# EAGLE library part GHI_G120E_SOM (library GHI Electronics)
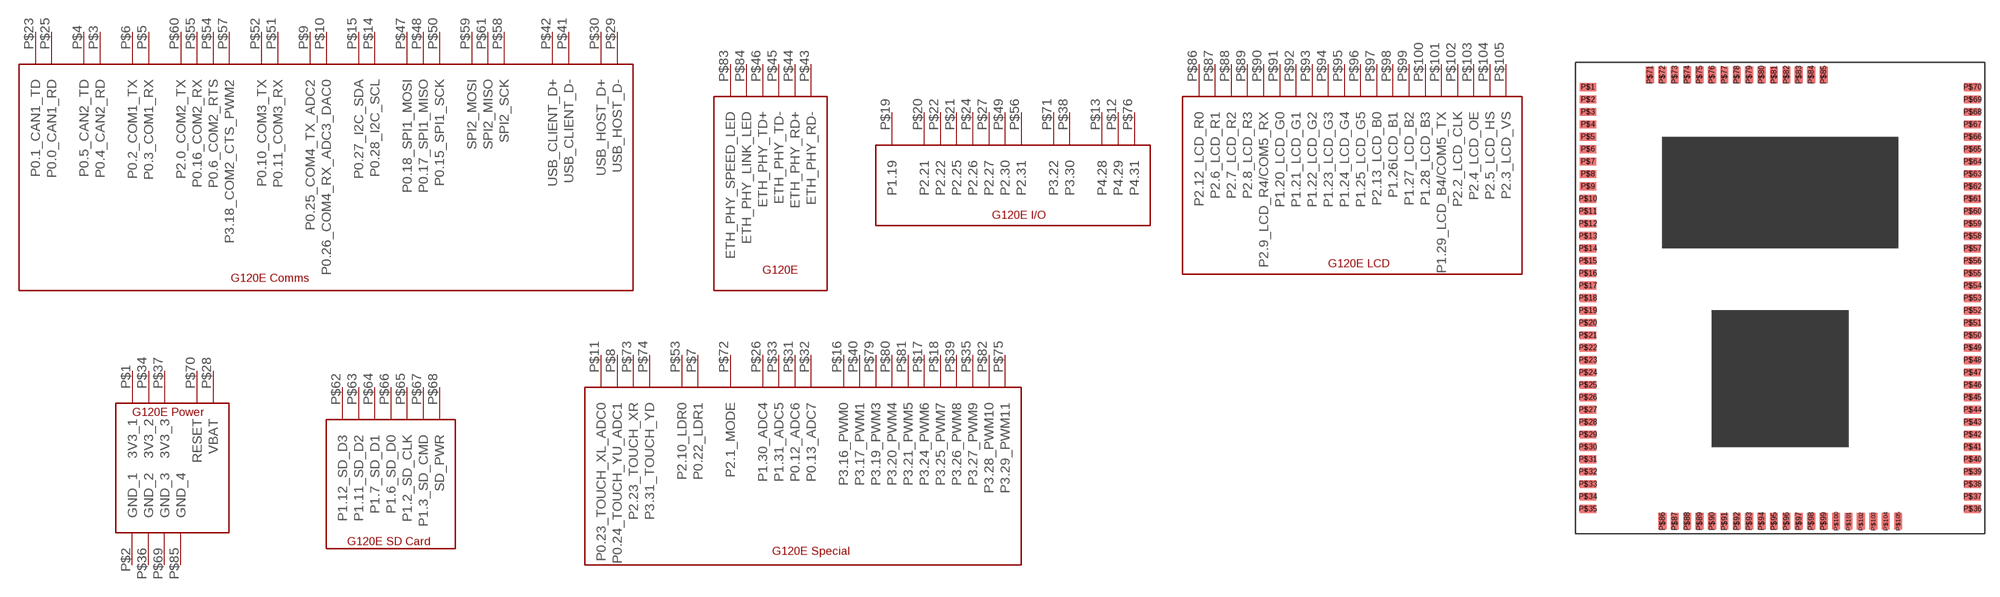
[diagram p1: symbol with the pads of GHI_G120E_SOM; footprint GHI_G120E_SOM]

Designator prefix -; gates G$1=GHI_G120E_COMMS G$2=GHI_G120E_ETH G$3=GHI_G120E_IO G$4=GHI_G120E_LCD G$5=GHI_G120E_PWR G$6=GHI_G120E_SD G$7=GHI_G120E_SPECIAL

## GHI_G120E_SOM  [GHI_G120E_SOM]
P$1  G$5:3V3_1
P$2  G$5:GND_1
P$3  G$1:P0.4_CAN2_RD
P$4  G$1:P0.5_CAN2_TD
P$5  G$1:P0.3_COM1_RX
P$6  G$1:P0.2_COM1_TX
P$7  G$7:P0.22_LDR1
P$8  G$7:P0.24_TOUCH_YU_ADC1
P$9  G$1:P0.25_COM4_TX_ADC2
P$10  G$1:P0.26_COM4_RX_ADC3_DAC0
P$11  G$7:P0.23_TOUCH_XL_ADC0
P$12  G$3:P4.29
P$13  G$3:P4.28
P$14  G$1:P0.28_I2C_SCL
P$15  G$1:P0.27_I2C_SDA
P$16  G$7:P3.16_PWM0
P$17  G$7:P3.24_PWM6
P$18  G$7:P3.25_PWM7
P$19  G$3:P1.19
P$20  G$3:P2.21
P$21  G$3:P2.25
P$22  G$3:P2.22
P$23  G$1:P0.1_CAN1_TD
P$24  G$3:P2.26
P$25  G$1:P0.0_CAN1_RD
P$26  G$7:P1.30_ADC4
P$27  G$3:P2.27
P$28  G$5:VBAT
P$29  G$1:USB_HOST_D-
P$30  G$1:USB_HOST_D+
P$31  G$7:P0.12_ADC6
P$32  G$7:P0.13_ADC7
P$33  G$7:P1.31_ADC5
P$34  G$5:3V3_2
P$35  G$7:P3.27_PWM9
P$36  G$5:GND_2
P$37  G$5:3V3_3
P$38  G$3:P3.30
P$39  G$7:P3.26_PWM8
P$40  G$7:P3.17_PWM1
P$41  G$1:USB_CLIENT_D-
P$42  G$1:USB_CLIENT_D+
P$43  G$2:ETH_PHY_RD-
P$44  G$2:ETH_PHY_RD+
P$45  G$2:ETH_PHY_TD-
P$46  G$2:ETH_PHY_TD+
P$47  G$1:P0.18_SPI1_MOSI
P$48  G$1:P0.17_SPI1_MISO
P$49  G$3:P2.30
P$50  G$1:P0.15_SPI1_SCK
P$51  G$1:P0.11_COM3_RX
P$52  G$1:P0.10_COM3_TX
P$53  G$7:P2.10_LDR0
P$54  G$1:P0.6_COM2_RTS
P$55  G$1:P0.16_COM2_RX
P$56  G$3:P2.31
P$57  G$1:P3.18_COM2_CTS_PWM2
P$58  G$1:SPI2_SCK
P$59  G$1:SPI2_MOSI
P$60  G$1:P2.0_COM2_TX
P$61  G$1:SPI2_MISO
P$62  G$6:P1.12_SD_D3
P$63  G$6:P1.11_SD_D2
P$64  G$6:P1.7_SD_D1
P$65  G$6:P1.2_SD_CLK
P$66  G$6:P1.6_SD_D0
P$67  G$6:P1.3_SD_CMD
P$68  G$6:SD_PWR
P$69  G$5:GND_3
P$70  G$5:RESET
P$71  G$3:P3.22
P$72  G$7:P2.1_MODE
P$73  G$7:P2.23_TOUCH_XR
P$74  G$7:P3.31_TOUCH_YD
P$75  G$7:P3.29_PWM11
P$76  G$3:P4.31
P$79  G$7:P3.19_PWM3
P$80  G$7:P3.20_PWM4
P$81  G$7:P3.21_PWM5
P$82  G$7:P3.28_PWM10
P$83  G$2:ETH_PHY_SPEED_LED
P$84  G$2:ETH_PHY_LINK_LED
P$85  G$5:GND_4
P$86  G$4:P2.12_LCD_R0
P$87  G$4:P2.6_LCD_R1
P$88  G$4:P2.7_LCD_R2
P$89  G$4:P2.8_LCD_R3
P$90  G$4:P2.9_LCD_R4/COM5_RX
P$91  G$4:P1.20_LCD_G0
P$92  G$4:P1.21_LCD_G1
P$93  G$4:P1.22_LCD_G2
P$94  G$4:P1.23_LCD_G3
P$95  G$4:P1.24_LCD_G4
P$96  G$4:P1.25_LCD_G5
P$97  G$4:P2.13_LCD_B0
P$98  G$4:P1.26LCD_B1
P$99  G$4:P1.27_LCD_B2
P$100  G$4:P1.28_LCD_B3
P$101  G$4:P1.29_LCD_B4/COM5_TX
P$102  G$4:P2.2_LCD_CLK
P$103  G$4:P2.4_LCD_OE
P$104  G$4:P2.5_LCD_HS
P$105  G$4:P2.3_LCD_VS

## Footprint GHI_G120E_SOM (pad centres in mm)
smd 1.676 x 0.813: P$1 -19.05,20.32; P$2 -19.05,19.05; P$3 -19.05,17.78; P$4 -19.05,16.51; P$5 -19.05,15.24; P$6 -19.05,13.97; P$7 -19.05,12.7; P$8 -19.05,11.43; P$9 -19.05,10.16; P$10 -19.05,8.89; P$11 -19.05,7.62; P$12 -19.05,6.35; P$13 -19.05,5.08; P$14 -19.05,3.81; P$15 -19.05,2.54; P$16 -19.05,1.27; P$17 -19.05,0; P$18 -19.05,-1.27; P$19 -19.05,-2.54; P$20 -19.05,-3.81; P$21 -19.05,-5.08; P$22 -19.05,-6.35; P$23 -19.05,-7.62; P$24 -19.05,-8.89; P$25 -19.05,-10.16; P$26 -19.05,-11.43; P$27 -19.05,-12.7; P$28 -19.05,-13.97; P$29 -19.05,-15.24; P$30 -19.05,-16.51; P$31 -19.05,-17.78; P$32 -19.05,-19.05; P$33 -19.05,-20.32; P$34 -19.05,-21.59; P$35 -19.05,-22.86; P$36 20.32,-22.86; P$37 20.32,-21.59; P$38 20.32,-20.32; P$39 20.32,-19.05; P$40 20.32,-17.78; P$41 20.32,-16.51; P$42 20.32,-15.24; P$43 20.32,-13.97; P$44 20.32,-12.7; P$45 20.32,-11.43; P$46 20.32,-10.16; P$47 20.32,-8.89; P$48 20.32,-7.62; P$49 20.32,-6.35; P$50 20.32,-5.08; P$51 20.32,-3.81; P$52 20.32,-2.54; P$53 20.32,-1.27; P$54 20.32,0; P$55 20.32,1.27; P$56 20.32,2.54; P$57 20.32,3.81; P$58 20.32,5.08; P$59 20.32,6.35; P$60 20.32,7.62; P$61 20.32,8.89; P$62 20.32,10.16; P$63 20.32,11.43; P$64 20.32,12.7; P$65 20.32,13.97; P$66 20.32,15.24; P$67 20.32,16.51; P$68 20.32,17.78; P$69 20.32,19.05; P$70 20.32,20.32
smd 0.813 x 1.676: P$71 -12.7,21.59; P$72 -11.43,21.59; P$73 -10.16,21.59; P$74 -8.89,21.59; P$75 -7.62,21.59; P$76 -6.35,21.59; P$77 -5.08,21.59; P$78 -3.81,21.59; P$79 -2.54,21.59; P$80 -1.27,21.59; P$81 0,21.59; P$82 1.27,21.59; P$83 2.54,21.59; P$84 3.81,21.59; P$85 5.08,21.59; P$86 -11.43,-24.13; P$87 -10.16,-24.13; P$88 -8.89,-24.13; P$89 -7.62,-24.13; P$90 -6.35,-24.13; P$91 -5.08,-24.13; P$92 -3.81,-24.13; P$93 -2.54,-24.13; P$94 -1.27,-24.13; P$95 0,-24.13; P$96 1.27,-24.13; P$97 2.54,-24.13; P$98 3.81,-24.13; P$99 5.08,-24.13; P$100 6.35,-24.13; P$101 7.62,-24.13; P$102 8.89,-24.13; P$103 10.16,-24.13; P$104 11.43,-24.13; P$105 12.7,-24.13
